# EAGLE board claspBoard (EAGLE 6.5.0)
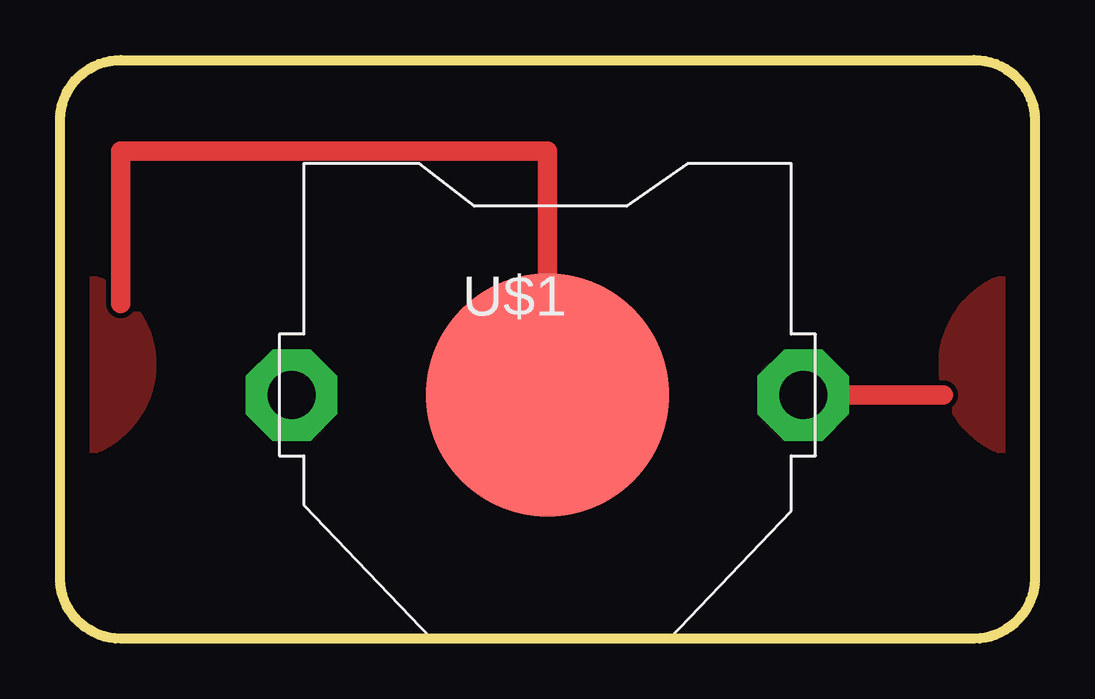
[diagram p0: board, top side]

Size 40.64 x 24.13 mm. Coordinates in mm from the lower left corner, seen from the top.
Outline: 0,2.54 0,21.59 arc-90 2.54,24.13 38.1,24.13 arc-90 40.64,21.59 40.64,2.54 arc-90 38.1,0 2.54,0 arc-90 0,2.54
Copper layers (1*16): Top 0.035mm / dielectric 1.5mm / Bottom 0.035mm
Design rules "default": minimum track width 10mil, minimum drill 24mil, track to track 8mil, track to pad 8mil, pad to pad 8mil, via to via 8mil, smd to smd 8mil, copper to edge 40mil, drill to drill 8mil, minimum pad ring 10mil, minimum via ring 8mil, stop-mask expansion 4mil, vias tented up to drill 0mil, thermal gap 10mil

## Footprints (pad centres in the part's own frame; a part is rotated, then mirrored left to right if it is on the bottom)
CR2032-THRU = drill 2 pad 3.81 octagon: +1 -10.668,0; +2 10.668,0 | smd 10.16 x 10.16: - 0,0

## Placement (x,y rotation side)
U$1  [CR2032-THRU]  20.32,10.16 0 top

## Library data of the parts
U$1 = adafruit

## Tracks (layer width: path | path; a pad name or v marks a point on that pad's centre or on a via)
N$1
  Top 0.813: 20.32,13.97 20.32,20.32 2.54,20.32 2.54,13.97
N$2
  pour Top: 0,15.24 arc-90 3.81,11.43 arc-90 0,7.62
  pour Top: 40.64,7.62 arc-90 36.83,11.43 arc-90 40.64,15.24
N$3
  Top 0.813: 30.48,10.16 36.83,10.16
